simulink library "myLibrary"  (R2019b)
settings: Solver=VariableStepAuto  StartTime=0.0  StopTime=10.0  RelTol=1e-3
undefined symbols (not defined in the file or in its folder): batt_delay, Calculation, cap_1ph, cap_3ph, Complex, Current, Dynamic, EV, ev_charger, EV_ID, ev_num, gcbh, Iabc, Load, max_charge_1ph, max_charge_3ph, max_disch_1ph, max_disch_3ph, MV_LV_transf, myLibrary, phase, Phase, Phasor, rated_1ph, rated_3ph, Single, SoC_init, SPDL, sps_rtmsupport, Tr_capacity, Tstep, Vabc, Vnom, yes
libraries: powerlib x163, $bdroot x13, spsVIMeasurementModel x3, simulink x2, powerlib_meascontrol x1
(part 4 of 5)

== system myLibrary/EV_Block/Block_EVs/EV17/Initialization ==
  Constant : Constant  Value=207.85
  Constant1 : Constant  Value=-120
  Constant2 : Constant  Value=-207.85
  Constant3 : Constant  Value=-120
  Constant4 : Constant  Value=0
  Constant5 : Constant  Value=240
  Constant6 : Constant  Value=Phase
  Data Type Conversion : DataTypeConversion  OutDataTypeStr=double
  Demux : Demux  Outputs=2
  If : If  IfExpression=u1 == 1  ElseIfExpressions=u1 == 2
  If Action Subsystem : Subsystem  TreatAsAtomicUnit=on
  If Action Subsystem1 : Subsystem  TreatAsAtomicUnit=on
  If Action Subsystem2 : Subsystem  TreatAsAtomicUnit=on
  Logical Operator : Logic  Operator=NOT  AllPortsSameDT=off  OutDataTypeStr=boolean
  Mux : Mux  Inputs=2
  Real-Imag to Complex : RealImagToComplex
  Real-Imag to Complex1 : RealImagToComplex
  Real-Imag to Complex2 : RealImagToComplex
  Switch : Switch  Criteria=u2 > Threshold
  Switch1 : Switch  Criteria=u2 > Threshold
  Out1 : Outport  VectorParamsAs1DForOutWhenUnconnected=off
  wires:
  Data Type Conversion/1 -> Mux/2
  [control] -> Demux/1
  Logical Operator/1 -> Data Type Conversion/1
  If Action Subsystem/1(Out1) -> Mux/1
  Mux/1 -> [control]
  If Action Subsystem2/1(Out1) -> Logical Operator/1
  Demux/2 -> Switch1/2
  Demux/1 -> Switch/2
  If/3 -> If Action Subsystem2/Action
  If/2 -> If Action Subsystem1/Action
  If/1 -> If Action Subsystem/Action
  Constant6/1 -> If/1
  Switch1/1 -> Out1/1
  Real-Imag to Complex2/1 -> Switch1/3
  Switch/1 -> Switch1/1
  Real-Imag to Complex1/1 -> Switch/3
  Real-Imag to Complex/1 -> Switch/1
  Constant4/1 -> Real-Imag to Complex2/1
  Constant5/1 -> Real-Imag to Complex2/2
  Constant2/1 -> Real-Imag to Complex1/1
  Constant3/1 -> Real-Imag to Complex1/2
  Constant/1 -> Real-Imag to Complex/1
  Constant1/1 -> Real-Imag to Complex/2

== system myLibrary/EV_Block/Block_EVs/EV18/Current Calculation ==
  Vp : Inport
  Constant : Constant  Commented=on  Value=2060
  Constant1 : Constant  Commented=on  Value=600
  Demux : Demux  Outputs=2
  Divide : Product  Inputs=*/
  From Workspace : FromWorkspace  VariableName=Load_Profile  SampleTime=0  OutputAfterFinalValue=Holding final value
  Gain : Gain  Gain=2
  Math Function : Math  Operator=conj
  Real-Imag to Complex : RealImagToComplex
  Isignal : Outport  VectorParamsAs1DForOutWhenUnconnected=off
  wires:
  Demux/2 -> Real-Imag to Complex/2
  Demux/1 -> Real-Imag to Complex/1
  Math Function/1 -> Isignal/1
  Divide/1 -> Math Function/1
  Gain/1 -> Divide/1
  Vp/1 -> Divide/2
  Real-Imag to Complex/1 -> Gain/1
  From Workspace/1 -> Demux/1

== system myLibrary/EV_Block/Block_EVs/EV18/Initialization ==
  Constant : Constant  Value=207.85
  Constant1 : Constant  Value=-120
  Constant2 : Constant  Value=-207.85
  Constant3 : Constant  Value=-120
  Constant4 : Constant  Value=0
  Constant5 : Constant  Value=240
  Constant6 : Constant  Value=Phase
  Data Type Conversion : DataTypeConversion  OutDataTypeStr=double
  Demux : Demux  Outputs=2
  If : If  IfExpression=u1 == 1  ElseIfExpressions=u1 == 2
  If Action Subsystem : Subsystem  TreatAsAtomicUnit=on
  If Action Subsystem1 : Subsystem  TreatAsAtomicUnit=on
  If Action Subsystem2 : Subsystem  TreatAsAtomicUnit=on
  Logical Operator : Logic  Operator=NOT  AllPortsSameDT=off  OutDataTypeStr=boolean
  Mux : Mux  Inputs=2
  Real-Imag to Complex : RealImagToComplex
  Real-Imag to Complex1 : RealImagToComplex
  Real-Imag to Complex2 : RealImagToComplex
  Switch : Switch  Criteria=u2 > Threshold
  Switch1 : Switch  Criteria=u2 > Threshold
  Out1 : Outport  VectorParamsAs1DForOutWhenUnconnected=off
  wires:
  Data Type Conversion/1 -> Mux/2
  [control] -> Demux/1
  Logical Operator/1 -> Data Type Conversion/1
  If Action Subsystem/1(Out1) -> Mux/1
  Mux/1 -> [control]
  If Action Subsystem2/1(Out1) -> Logical Operator/1
  Demux/2 -> Switch1/2
  Demux/1 -> Switch/2
  If/3 -> If Action Subsystem2/Action
  If/2 -> If Action Subsystem1/Action
  If/1 -> If Action Subsystem/Action
  Constant6/1 -> If/1
  Switch1/1 -> Out1/1
  Real-Imag to Complex2/1 -> Switch1/3
  Switch/1 -> Switch1/1
  Real-Imag to Complex1/1 -> Switch/3
  Real-Imag to Complex/1 -> Switch/1
  Constant4/1 -> Real-Imag to Complex2/1
  Constant5/1 -> Real-Imag to Complex2/2
  Constant2/1 -> Real-Imag to Complex1/1
  Constant3/1 -> Real-Imag to Complex1/2
  Constant/1 -> Real-Imag to Complex/1
  Constant1/1 -> Real-Imag to Complex/2

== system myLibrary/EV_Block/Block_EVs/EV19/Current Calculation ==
  Vp : Inport
  Constant : Constant  Commented=on  Value=2060
  Constant1 : Constant  Commented=on  Value=600
  Demux : Demux  Outputs=2
  Divide : Product  Inputs=*/
  From Workspace : FromWorkspace  VariableName=Load_Profile  SampleTime=0  OutputAfterFinalValue=Holding final value
  Gain : Gain  Gain=2
  Math Function : Math  Operator=conj
  Real-Imag to Complex : RealImagToComplex
  Isignal : Outport  VectorParamsAs1DForOutWhenUnconnected=off
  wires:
  Demux/2 -> Real-Imag to Complex/2
  Demux/1 -> Real-Imag to Complex/1
  Math Function/1 -> Isignal/1
  Divide/1 -> Math Function/1
  Gain/1 -> Divide/1
  Vp/1 -> Divide/2
  Real-Imag to Complex/1 -> Gain/1
  From Workspace/1 -> Demux/1

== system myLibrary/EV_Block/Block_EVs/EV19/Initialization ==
  Constant : Constant  Value=207.85
  Constant1 : Constant  Value=-120
  Constant2 : Constant  Value=-207.85
  Constant3 : Constant  Value=-120
  Constant4 : Constant  Value=0
  Constant5 : Constant  Value=240
  Constant6 : Constant  Value=Phase
  Data Type Conversion : DataTypeConversion  OutDataTypeStr=double
  Demux : Demux  Outputs=2
  If : If  IfExpression=u1 == 1  ElseIfExpressions=u1 == 2
  If Action Subsystem : Subsystem  TreatAsAtomicUnit=on
  If Action Subsystem1 : Subsystem  TreatAsAtomicUnit=on
  If Action Subsystem2 : Subsystem  TreatAsAtomicUnit=on
  Logical Operator : Logic  Operator=NOT  AllPortsSameDT=off  OutDataTypeStr=boolean
  Mux : Mux  Inputs=2
  Real-Imag to Complex : RealImagToComplex
  Real-Imag to Complex1 : RealImagToComplex
  Real-Imag to Complex2 : RealImagToComplex
  Switch : Switch  Criteria=u2 > Threshold
  Switch1 : Switch  Criteria=u2 > Threshold
  Out1 : Outport  VectorParamsAs1DForOutWhenUnconnected=off
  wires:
  Data Type Conversion/1 -> Mux/2
  [control] -> Demux/1
  Logical Operator/1 -> Data Type Conversion/1
  If Action Subsystem/1(Out1) -> Mux/1
  Mux/1 -> [control]
  If Action Subsystem2/1(Out1) -> Logical Operator/1
  Demux/2 -> Switch1/2
  Demux/1 -> Switch/2
  If/3 -> If Action Subsystem2/Action
  If/2 -> If Action Subsystem1/Action
  If/1 -> If Action Subsystem/Action
  Constant6/1 -> If/1
  Switch1/1 -> Out1/1
  Real-Imag to Complex2/1 -> Switch1/3
  Switch/1 -> Switch1/1
  Real-Imag to Complex1/1 -> Switch/3
  Real-Imag to Complex/1 -> Switch/1
  Constant4/1 -> Real-Imag to Complex2/1
  Constant5/1 -> Real-Imag to Complex2/2
  Constant2/1 -> Real-Imag to Complex1/1
  Constant3/1 -> Real-Imag to Complex1/2
  Constant/1 -> Real-Imag to Complex/1
  Constant1/1 -> Real-Imag to Complex/2

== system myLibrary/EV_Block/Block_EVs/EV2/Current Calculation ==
  Vp : Inport
  Constant : Constant  Commented=on  Value=2060
  Constant1 : Constant  Commented=on  Value=600
  Demux : Demux  Outputs=2
  Divide : Product  Inputs=*/
  From Workspace : FromWorkspace  VariableName=Load_Profile  SampleTime=0  OutputAfterFinalValue=Holding final value
  Gain : Gain  Gain=2
  Math Function : Math  Operator=conj
  Real-Imag to Complex : RealImagToComplex
  Isignal : Outport  VectorParamsAs1DForOutWhenUnconnected=off
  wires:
  Demux/2 -> Real-Imag to Complex/2
  Demux/1 -> Real-Imag to Complex/1
  Math Function/1 -> Isignal/1
  Divide/1 -> Math Function/1
  Gain/1 -> Divide/1
  Vp/1 -> Divide/2
  Real-Imag to Complex/1 -> Gain/1
  From Workspace/1 -> Demux/1

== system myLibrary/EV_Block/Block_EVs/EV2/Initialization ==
  Constant : Constant  Value=207.85
  Constant1 : Constant  Value=-120
  Constant2 : Constant  Value=-207.85
  Constant3 : Constant  Value=-120
  Constant4 : Constant  Value=0
  Constant5 : Constant  Value=240
  Constant6 : Constant  Value=Phase
  Data Type Conversion : DataTypeConversion  OutDataTypeStr=double
  Demux : Demux  Outputs=2
  If : If  IfExpression=u1 == 1  ElseIfExpressions=u1 == 2
  If Action Subsystem : Subsystem  TreatAsAtomicUnit=on
  If Action Subsystem1 : Subsystem  TreatAsAtomicUnit=on
  If Action Subsystem2 : Subsystem  TreatAsAtomicUnit=on
  Logical Operator : Logic  Operator=NOT  AllPortsSameDT=off  OutDataTypeStr=boolean
  Mux : Mux  Inputs=2
  Real-Imag to Complex : RealImagToComplex
  Real-Imag to Complex1 : RealImagToComplex
  Real-Imag to Complex2 : RealImagToComplex
  Switch : Switch  Criteria=u2 > Threshold
  Switch1 : Switch  Criteria=u2 > Threshold
  Out1 : Outport  VectorParamsAs1DForOutWhenUnconnected=off
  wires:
  Data Type Conversion/1 -> Mux/2
  [control] -> Demux/1
  Logical Operator/1 -> Data Type Conversion/1
  If Action Subsystem/1(Out1) -> Mux/1
  Mux/1 -> [control]
  If Action Subsystem2/1(Out1) -> Logical Operator/1
  Demux/2 -> Switch1/2
  Demux/1 -> Switch/2
  If/3 -> If Action Subsystem2/Action
  If/2 -> If Action Subsystem1/Action
  If/1 -> If Action Subsystem/Action
  Constant6/1 -> If/1
  Switch1/1 -> Out1/1
  Real-Imag to Complex2/1 -> Switch1/3
  Switch/1 -> Switch1/1
  Real-Imag to Complex1/1 -> Switch/3
  Real-Imag to Complex/1 -> Switch/1
  Constant4/1 -> Real-Imag to Complex2/1
  Constant5/1 -> Real-Imag to Complex2/2
  Constant2/1 -> Real-Imag to Complex1/1
  Constant3/1 -> Real-Imag to Complex1/2
  Constant/1 -> Real-Imag to Complex/1
  Constant1/1 -> Real-Imag to Complex/2

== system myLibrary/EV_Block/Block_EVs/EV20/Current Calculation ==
  Vp : Inport
  Constant : Constant  Commented=on  Value=2060
  Constant1 : Constant  Commented=on  Value=600
  Demux : Demux  Outputs=2
  Divide : Product  Inputs=*/
  From Workspace : FromWorkspace  VariableName=Load_Profile  SampleTime=0  OutputAfterFinalValue=Holding final value
  Gain : Gain  Gain=2
  Math Function : Math  Operator=conj
  Real-Imag to Complex : RealImagToComplex
  Isignal : Outport  VectorParamsAs1DForOutWhenUnconnected=off
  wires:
  Demux/2 -> Real-Imag to Complex/2
  Demux/1 -> Real-Imag to Complex/1
  Math Function/1 -> Isignal/1
  Divide/1 -> Math Function/1
  Gain/1 -> Divide/1
  Vp/1 -> Divide/2
  Real-Imag to Complex/1 -> Gain/1
  From Workspace/1 -> Demux/1

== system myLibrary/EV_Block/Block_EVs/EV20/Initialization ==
  Constant : Constant  Value=207.85
  Constant1 : Constant  Value=-120
  Constant2 : Constant  Value=-207.85
  Constant3 : Constant  Value=-120
  Constant4 : Constant  Value=0
  Constant5 : Constant  Value=240
  Constant6 : Constant  Value=Phase
  Data Type Conversion : DataTypeConversion  OutDataTypeStr=double
  Demux : Demux  Outputs=2
  If : If  IfExpression=u1 == 1  ElseIfExpressions=u1 == 2
  If Action Subsystem : Subsystem  TreatAsAtomicUnit=on
  If Action Subsystem1 : Subsystem  TreatAsAtomicUnit=on
  If Action Subsystem2 : Subsystem  TreatAsAtomicUnit=on
  Logical Operator : Logic  Operator=NOT  AllPortsSameDT=off  OutDataTypeStr=boolean
  Mux : Mux  Inputs=2
  Real-Imag to Complex : RealImagToComplex
  Real-Imag to Complex1 : RealImagToComplex
  Real-Imag to Complex2 : RealImagToComplex
  Switch : Switch  Criteria=u2 > Threshold
  Switch1 : Switch  Criteria=u2 > Threshold
  Out1 : Outport  VectorParamsAs1DForOutWhenUnconnected=off
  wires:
  Data Type Conversion/1 -> Mux/2
  [control] -> Demux/1
  Logical Operator/1 -> Data Type Conversion/1
  If Action Subsystem/1(Out1) -> Mux/1
  Mux/1 -> [control]
  If Action Subsystem2/1(Out1) -> Logical Operator/1
  Demux/2 -> Switch1/2
  Demux/1 -> Switch/2
  If/3 -> If Action Subsystem2/Action
  If/2 -> If Action Subsystem1/Action
  If/1 -> If Action Subsystem/Action
  Constant6/1 -> If/1
  Switch1/1 -> Out1/1
  Real-Imag to Complex2/1 -> Switch1/3
  Switch/1 -> Switch1/1
  Real-Imag to Complex1/1 -> Switch/3
  Real-Imag to Complex/1 -> Switch/1
  Constant4/1 -> Real-Imag to Complex2/1
  Constant5/1 -> Real-Imag to Complex2/2
  Constant2/1 -> Real-Imag to Complex1/1
  Constant3/1 -> Real-Imag to Complex1/2
  Constant/1 -> Real-Imag to Complex/1
  Constant1/1 -> Real-Imag to Complex/2

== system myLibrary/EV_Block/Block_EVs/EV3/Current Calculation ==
  Vp : Inport
  Constant : Constant  Commented=on  Value=2060
  Constant1 : Constant  Commented=on  Value=600
  Demux : Demux  Outputs=2
  Divide : Product  Inputs=*/
  From Workspace : FromWorkspace  VariableName=Load_Profile  SampleTime=0  OutputAfterFinalValue=Holding final value
  Gain : Gain  Gain=2
  Math Function : Math  Operator=conj
  Real-Imag to Complex : RealImagToComplex
  Isignal : Outport  VectorParamsAs1DForOutWhenUnconnected=off
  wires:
  Demux/2 -> Real-Imag to Complex/2
  Demux/1 -> Real-Imag to Complex/1
  Math Function/1 -> Isignal/1
  Divide/1 -> Math Function/1
  Gain/1 -> Divide/1
  Vp/1 -> Divide/2
  Real-Imag to Complex/1 -> Gain/1
  From Workspace/1 -> Demux/1

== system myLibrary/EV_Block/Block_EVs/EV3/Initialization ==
  Constant : Constant  Value=207.85
  Constant1 : Constant  Value=-120
  Constant2 : Constant  Value=-207.85
  Constant3 : Constant  Value=-120
  Constant4 : Constant  Value=0
  Constant5 : Constant  Value=240
  Constant6 : Constant  Value=Phase
  Data Type Conversion : DataTypeConversion  OutDataTypeStr=double
  Demux : Demux  Outputs=2
  If : If  IfExpression=u1 == 1  ElseIfExpressions=u1 == 2
  If Action Subsystem : Subsystem  TreatAsAtomicUnit=on
  If Action Subsystem1 : Subsystem  TreatAsAtomicUnit=on
  If Action Subsystem2 : Subsystem  TreatAsAtomicUnit=on
  Logical Operator : Logic  Operator=NOT  AllPortsSameDT=off  OutDataTypeStr=boolean
  Mux : Mux  Inputs=2
  Real-Imag to Complex : RealImagToComplex
  Real-Imag to Complex1 : RealImagToComplex
  Real-Imag to Complex2 : RealImagToComplex
  Switch : Switch  Criteria=u2 > Threshold
  Switch1 : Switch  Criteria=u2 > Threshold
  Out1 : Outport  VectorParamsAs1DForOutWhenUnconnected=off
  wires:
  Data Type Conversion/1 -> Mux/2
  [control] -> Demux/1
  Logical Operator/1 -> Data Type Conversion/1
  If Action Subsystem/1(Out1) -> Mux/1
  Mux/1 -> [control]
  If Action Subsystem2/1(Out1) -> Logical Operator/1
  Demux/2 -> Switch1/2
  Demux/1 -> Switch/2
  If/3 -> If Action Subsystem2/Action
  If/2 -> If Action Subsystem1/Action
  If/1 -> If Action Subsystem/Action
  Constant6/1 -> If/1
  Switch1/1 -> Out1/1
  Real-Imag to Complex2/1 -> Switch1/3
  Switch/1 -> Switch1/1
  Real-Imag to Complex1/1 -> Switch/3
  Real-Imag to Complex/1 -> Switch/1
  Constant4/1 -> Real-Imag to Complex2/1
  Constant5/1 -> Real-Imag to Complex2/2
  Constant2/1 -> Real-Imag to Complex1/1
  Constant3/1 -> Real-Imag to Complex1/2
  Constant/1 -> Real-Imag to Complex/1
  Constant1/1 -> Real-Imag to Complex/2

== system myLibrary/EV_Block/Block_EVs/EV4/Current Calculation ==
  Vp : Inport
  Constant : Constant  Commented=on  Value=2060
  Constant1 : Constant  Commented=on  Value=600
  Demux : Demux  Outputs=2
  Divide : Product  Inputs=*/
  From Workspace : FromWorkspace  VariableName=Load_Profile  SampleTime=0  OutputAfterFinalValue=Holding final value
  Gain : Gain  Gain=2
  Math Function : Math  Operator=conj
  Real-Imag to Complex : RealImagToComplex
  Isignal : Outport  VectorParamsAs1DForOutWhenUnconnected=off
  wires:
  Demux/2 -> Real-Imag to Complex/2
  Demux/1 -> Real-Imag to Complex/1
  Math Function/1 -> Isignal/1
  Divide/1 -> Math Function/1
  Gain/1 -> Divide/1
  Vp/1 -> Divide/2
  Real-Imag to Complex/1 -> Gain/1
  From Workspace/1 -> Demux/1

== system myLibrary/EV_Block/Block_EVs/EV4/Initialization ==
  Constant : Constant  Value=207.85
  Constant1 : Constant  Value=-120
  Constant2 : Constant  Value=-207.85
  Constant3 : Constant  Value=-120
  Constant4 : Constant  Value=0
  Constant5 : Constant  Value=240
  Constant6 : Constant  Value=Phase
  Data Type Conversion : DataTypeConversion  OutDataTypeStr=double
  Demux : Demux  Outputs=2
  If : If  IfExpression=u1 == 1  ElseIfExpressions=u1 == 2
  If Action Subsystem : Subsystem  TreatAsAtomicUnit=on
  If Action Subsystem1 : Subsystem  TreatAsAtomicUnit=on
  If Action Subsystem2 : Subsystem  TreatAsAtomicUnit=on
  Logical Operator : Logic  Operator=NOT  AllPortsSameDT=off  OutDataTypeStr=boolean
  Mux : Mux  Inputs=2
  Real-Imag to Complex : RealImagToComplex
  Real-Imag to Complex1 : RealImagToComplex
  Real-Imag to Complex2 : RealImagToComplex
  Switch : Switch  Criteria=u2 > Threshold
  Switch1 : Switch  Criteria=u2 > Threshold
  Out1 : Outport  VectorParamsAs1DForOutWhenUnconnected=off
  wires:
  Data Type Conversion/1 -> Mux/2
  [control] -> Demux/1
  Logical Operator/1 -> Data Type Conversion/1
  If Action Subsystem/1(Out1) -> Mux/1
  Mux/1 -> [control]
  If Action Subsystem2/1(Out1) -> Logical Operator/1
  Demux/2 -> Switch1/2
  Demux/1 -> Switch/2
  If/3 -> If Action Subsystem2/Action
  If/2 -> If Action Subsystem1/Action
  If/1 -> If Action Subsystem/Action
  Constant6/1 -> If/1
  Switch1/1 -> Out1/1
  Real-Imag to Complex2/1 -> Switch1/3
  Switch/1 -> Switch1/1
  Real-Imag to Complex1/1 -> Switch/3
  Real-Imag to Complex/1 -> Switch/1
  Constant4/1 -> Real-Imag to Complex2/1
  Constant5/1 -> Real-Imag to Complex2/2
  Constant2/1 -> Real-Imag to Complex1/1
  Constant3/1 -> Real-Imag to Complex1/2
  Constant/1 -> Real-Imag to Complex/1
  Constant1/1 -> Real-Imag to Complex/2

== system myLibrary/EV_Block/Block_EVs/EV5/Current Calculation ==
  Vp : Inport
  Constant : Constant  Commented=on  Value=2060
  Constant1 : Constant  Commented=on  Value=600
  Demux : Demux  Outputs=2
  Divide : Product  Inputs=*/
  From Workspace : FromWorkspace  VariableName=Load_Profile  SampleTime=0  OutputAfterFinalValue=Holding final value
  Gain : Gain  Gain=2
  Math Function : Math  Operator=conj
  Real-Imag to Complex : RealImagToComplex
  Isignal : Outport  VectorParamsAs1DForOutWhenUnconnected=off
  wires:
  Demux/2 -> Real-Imag to Complex/2
  Demux/1 -> Real-Imag to Complex/1
  Math Function/1 -> Isignal/1
  Divide/1 -> Math Function/1
  Gain/1 -> Divide/1
  Vp/1 -> Divide/2
  Real-Imag to Complex/1 -> Gain/1
  From Workspace/1 -> Demux/1

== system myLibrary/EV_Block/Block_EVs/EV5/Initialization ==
  Constant : Constant  Value=207.85
  Constant1 : Constant  Value=-120
  Constant2 : Constant  Value=-207.85
  Constant3 : Constant  Value=-120
  Constant4 : Constant  Value=0
  Constant5 : Constant  Value=240
  Constant6 : Constant  Value=Phase
  Data Type Conversion : DataTypeConversion  OutDataTypeStr=double
  Demux : Demux  Outputs=2
  If : If  IfExpression=u1 == 1  ElseIfExpressions=u1 == 2
  If Action Subsystem : Subsystem  TreatAsAtomicUnit=on
  If Action Subsystem1 : Subsystem  TreatAsAtomicUnit=on
  If Action Subsystem2 : Subsystem  TreatAsAtomicUnit=on
  Logical Operator : Logic  Operator=NOT  AllPortsSameDT=off  OutDataTypeStr=boolean
  Mux : Mux  Inputs=2
  Real-Imag to Complex : RealImagToComplex
  Real-Imag to Complex1 : RealImagToComplex
  Real-Imag to Complex2 : RealImagToComplex
  Switch : Switch  Criteria=u2 > Threshold
  Switch1 : Switch  Criteria=u2 > Threshold
  Out1 : Outport  VectorParamsAs1DForOutWhenUnconnected=off
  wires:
  Data Type Conversion/1 -> Mux/2
  [control] -> Demux/1
  Logical Operator/1 -> Data Type Conversion/1
  If Action Subsystem/1(Out1) -> Mux/1
  Mux/1 -> [control]
  If Action Subsystem2/1(Out1) -> Logical Operator/1
  Demux/2 -> Switch1/2
  Demux/1 -> Switch/2
  If/3 -> If Action Subsystem2/Action
  If/2 -> If Action Subsystem1/Action
  If/1 -> If Action Subsystem/Action
  Constant6/1 -> If/1
  Switch1/1 -> Out1/1
  Real-Imag to Complex2/1 -> Switch1/3
  Switch/1 -> Switch1/1
  Real-Imag to Complex1/1 -> Switch/3
  Real-Imag to Complex/1 -> Switch/1
  Constant4/1 -> Real-Imag to Complex2/1
  Constant5/1 -> Real-Imag to Complex2/2
  Constant2/1 -> Real-Imag to Complex1/1
  Constant3/1 -> Real-Imag to Complex1/2
  Constant/1 -> Real-Imag to Complex/1
  Constant1/1 -> Real-Imag to Complex/2

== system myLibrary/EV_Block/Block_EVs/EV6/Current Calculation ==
  Vp : Inport
  Constant : Constant  Commented=on  Value=2060
  Constant1 : Constant  Commented=on  Value=600
  Demux : Demux  Outputs=2
  Divide : Product  Inputs=*/
  From Workspace : FromWorkspace  VariableName=Load_Profile  SampleTime=0  OutputAfterFinalValue=Holding final value
  Gain : Gain  Gain=2
  Math Function : Math  Operator=conj
  Real-Imag to Complex : RealImagToComplex
  Isignal : Outport  VectorParamsAs1DForOutWhenUnconnected=off
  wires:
  Demux/2 -> Real-Imag to Complex/2
  Demux/1 -> Real-Imag to Complex/1
  Math Function/1 -> Isignal/1
  Divide/1 -> Math Function/1
  Gain/1 -> Divide/1
  Vp/1 -> Divide/2
  Real-Imag to Complex/1 -> Gain/1
  From Workspace/1 -> Demux/1

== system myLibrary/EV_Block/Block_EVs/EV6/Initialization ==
  Constant : Constant  Value=207.85
  Constant1 : Constant  Value=-120
  Constant2 : Constant  Value=-207.85
  Constant3 : Constant  Value=-120
  Constant4 : Constant  Value=0
  Constant5 : Constant  Value=240
  Constant6 : Constant  Value=Phase
  Data Type Conversion : DataTypeConversion  OutDataTypeStr=double
  Demux : Demux  Outputs=2
  If : If  IfExpression=u1 == 1  ElseIfExpressions=u1 == 2
  If Action Subsystem : Subsystem  TreatAsAtomicUnit=on
  If Action Subsystem1 : Subsystem  TreatAsAtomicUnit=on
  If Action Subsystem2 : Subsystem  TreatAsAtomicUnit=on
  Logical Operator : Logic  Operator=NOT  AllPortsSameDT=off  OutDataTypeStr=boolean
  Mux : Mux  Inputs=2
  Real-Imag to Complex : RealImagToComplex
  Real-Imag to Complex1 : RealImagToComplex
  Real-Imag to Complex2 : RealImagToComplex
  Switch : Switch  Criteria=u2 > Threshold
  Switch1 : Switch  Criteria=u2 > Threshold
  Out1 : Outport  VectorParamsAs1DForOutWhenUnconnected=off
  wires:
  Data Type Conversion/1 -> Mux/2
  [control] -> Demux/1
  Logical Operator/1 -> Data Type Conversion/1
  If Action Subsystem/1(Out1) -> Mux/1
  Mux/1 -> [control]
  If Action Subsystem2/1(Out1) -> Logical Operator/1
  Demux/2 -> Switch1/2
  Demux/1 -> Switch/2
  If/3 -> If Action Subsystem2/Action
  If/2 -> If Action Subsystem1/Action
  If/1 -> If Action Subsystem/Action
  Constant6/1 -> If/1
  Switch1/1 -> Out1/1
  Real-Imag to Complex2/1 -> Switch1/3
  Switch/1 -> Switch1/1
  Real-Imag to Complex1/1 -> Switch/3
  Real-Imag to Complex/1 -> Switch/1
  Constant4/1 -> Real-Imag to Complex2/1
  Constant5/1 -> Real-Imag to Complex2/2
  Constant2/1 -> Real-Imag to Complex1/1
  Constant3/1 -> Real-Imag to Complex1/2
  Constant/1 -> Real-Imag to Complex/1
  Constant1/1 -> Real-Imag to Complex/2

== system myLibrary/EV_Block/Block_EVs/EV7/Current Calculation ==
  Vp : Inport
  Constant : Constant  Commented=on  Value=2060
  Constant1 : Constant  Commented=on  Value=600
  Demux : Demux  Outputs=2
  Divide : Product  Inputs=*/
  From Workspace : FromWorkspace  VariableName=Load_Profile  SampleTime=0  OutputAfterFinalValue=Holding final value
  Gain : Gain  Gain=2
  Math Function : Math  Operator=conj
  Real-Imag to Complex : RealImagToComplex
  Isignal : Outport  VectorParamsAs1DForOutWhenUnconnected=off
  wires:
  Demux/2 -> Real-Imag to Complex/2
  Demux/1 -> Real-Imag to Complex/1
  Math Function/1 -> Isignal/1
  Divide/1 -> Math Function/1
  Gain/1 -> Divide/1
  Vp/1 -> Divide/2
  Real-Imag to Complex/1 -> Gain/1
  From Workspace/1 -> Demux/1

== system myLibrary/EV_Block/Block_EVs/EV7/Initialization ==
  Constant : Constant  Value=207.85
  Constant1 : Constant  Value=-120
  Constant2 : Constant  Value=-207.85
  Constant3 : Constant  Value=-120
  Constant4 : Constant  Value=0
  Constant5 : Constant  Value=240
  Constant6 : Constant  Value=Phase
  Data Type Conversion : DataTypeConversion  OutDataTypeStr=double
  Demux : Demux  Outputs=2
  If : If  IfExpression=u1 == 1  ElseIfExpressions=u1 == 2
  If Action Subsystem : Subsystem  TreatAsAtomicUnit=on
  If Action Subsystem1 : Subsystem  TreatAsAtomicUnit=on
  If Action Subsystem2 : Subsystem  TreatAsAtomicUnit=on
  Logical Operator : Logic  Operator=NOT  AllPortsSameDT=off  OutDataTypeStr=boolean
  Mux : Mux  Inputs=2
  Real-Imag to Complex : RealImagToComplex
  Real-Imag to Complex1 : RealImagToComplex
  Real-Imag to Complex2 : RealImagToComplex
  Switch : Switch  Criteria=u2 > Threshold
  Switch1 : Switch  Criteria=u2 > Threshold
  Out1 : Outport  VectorParamsAs1DForOutWhenUnconnected=off
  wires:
  Data Type Conversion/1 -> Mux/2
  [control] -> Demux/1
  Logical Operator/1 -> Data Type Conversion/1
  If Action Subsystem/1(Out1) -> Mux/1
  Mux/1 -> [control]
  If Action Subsystem2/1(Out1) -> Logical Operator/1
  Demux/2 -> Switch1/2
  Demux/1 -> Switch/2
  If/3 -> If Action Subsystem2/Action
  If/2 -> If Action Subsystem1/Action
  If/1 -> If Action Subsystem/Action
  Constant6/1 -> If/1
  Switch1/1 -> Out1/1
  Real-Imag to Complex2/1 -> Switch1/3
  Switch/1 -> Switch1/1
  Real-Imag to Complex1/1 -> Switch/3
  Real-Imag to Complex/1 -> Switch/1
  Constant4/1 -> Real-Imag to Complex2/1
  Constant5/1 -> Real-Imag to Complex2/2
  Constant2/1 -> Real-Imag to Complex1/1
  Constant3/1 -> Real-Imag to Complex1/2
  Constant/1 -> Real-Imag to Complex/1
  Constant1/1 -> Real-Imag to Complex/2

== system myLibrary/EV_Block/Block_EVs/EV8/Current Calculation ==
  Vp : Inport
  Constant : Constant  Commented=on  Value=2060
  Constant1 : Constant  Commented=on  Value=600
  Demux : Demux  Outputs=2
  Divide : Product  Inputs=*/
  From Workspace : FromWorkspace  VariableName=Load_Profile  SampleTime=0  OutputAfterFinalValue=Holding final value
  Gain : Gain  Gain=2
  Math Function : Math  Operator=conj
  Real-Imag to Complex : RealImagToComplex
  Isignal : Outport  VectorParamsAs1DForOutWhenUnconnected=off
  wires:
  Demux/2 -> Real-Imag to Complex/2
  Demux/1 -> Real-Imag to Complex/1
  Math Function/1 -> Isignal/1
  Divide/1 -> Math Function/1
  Gain/1 -> Divide/1
  Vp/1 -> Divide/2
  Real-Imag to Complex/1 -> Gain/1
  From Workspace/1 -> Demux/1

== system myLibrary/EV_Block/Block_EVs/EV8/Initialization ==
  Constant : Constant  Value=207.85
  Constant1 : Constant  Value=-120
  Constant2 : Constant  Value=-207.85
  Constant3 : Constant  Value=-120
  Constant4 : Constant  Value=0
  Constant5 : Constant  Value=240
  Constant6 : Constant  Value=Phase
  Data Type Conversion : DataTypeConversion  OutDataTypeStr=double
  Demux : Demux  Outputs=2
  If : If  IfExpression=u1 == 1  ElseIfExpressions=u1 == 2
  If Action Subsystem : Subsystem  TreatAsAtomicUnit=on
  If Action Subsystem1 : Subsystem  TreatAsAtomicUnit=on
  If Action Subsystem2 : Subsystem  TreatAsAtomicUnit=on
  Logical Operator : Logic  Operator=NOT  AllPortsSameDT=off  OutDataTypeStr=boolean
  Mux : Mux  Inputs=2
  Real-Imag to Complex : RealImagToComplex
  Real-Imag to Complex1 : RealImagToComplex
  Real-Imag to Complex2 : RealImagToComplex
  Switch : Switch  Criteria=u2 > Threshold
  Switch1 : Switch  Criteria=u2 > Threshold
  Out1 : Outport  VectorParamsAs1DForOutWhenUnconnected=off
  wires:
  Data Type Conversion/1 -> Mux/2
  [control] -> Demux/1
  Logical Operator/1 -> Data Type Conversion/1
  If Action Subsystem/1(Out1) -> Mux/1
  Mux/1 -> [control]
  If Action Subsystem2/1(Out1) -> Logical Operator/1
  Demux/2 -> Switch1/2
  Demux/1 -> Switch/2
  If/3 -> If Action Subsystem2/Action
  If/2 -> If Action Subsystem1/Action
  If/1 -> If Action Subsystem/Action
  Constant6/1 -> If/1
  Switch1/1 -> Out1/1
  Real-Imag to Complex2/1 -> Switch1/3
  Switch/1 -> Switch1/1
  Real-Imag to Complex1/1 -> Switch/3
  Real-Imag to Complex/1 -> Switch/1
  Constant4/1 -> Real-Imag to Complex2/1
  Constant5/1 -> Real-Imag to Complex2/2
  Constant2/1 -> Real-Imag to Complex1/1
  Constant3/1 -> Real-Imag to Complex1/2
  Constant/1 -> Real-Imag to Complex/1
  Constant1/1 -> Real-Imag to Complex/2

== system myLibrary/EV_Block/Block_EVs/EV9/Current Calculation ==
  Vp : Inport
  Constant : Constant  Commented=on  Value=2060
  Constant1 : Constant  Commented=on  Value=600
  Demux : Demux  Outputs=2
  Divide : Product  Inputs=*/
  From Workspace : FromWorkspace  VariableName=Load_Profile  SampleTime=0  OutputAfterFinalValue=Holding final value
  Gain : Gain  Gain=2
  Math Function : Math  Operator=conj
  Real-Imag to Complex : RealImagToComplex
  Isignal : Outport  VectorParamsAs1DForOutWhenUnconnected=off
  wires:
  Demux/2 -> Real-Imag to Complex/2
  Demux/1 -> Real-Imag to Complex/1
  Math Function/1 -> Isignal/1
  Divide/1 -> Math Function/1
  Gain/1 -> Divide/1
  Vp/1 -> Divide/2
  Real-Imag to Complex/1 -> Gain/1
  From Workspace/1 -> Demux/1

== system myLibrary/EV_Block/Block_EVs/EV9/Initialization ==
  Constant : Constant  Value=207.85
  Constant1 : Constant  Value=-120
  Constant2 : Constant  Value=-207.85
  Constant3 : Constant  Value=-120
  Constant4 : Constant  Value=0
  Constant5 : Constant  Value=240
  Constant6 : Constant  Value=Phase
  Data Type Conversion : DataTypeConversion  OutDataTypeStr=double
  Demux : Demux  Outputs=2
  If : If  IfExpression=u1 == 1  ElseIfExpressions=u1 == 2
  If Action Subsystem : Subsystem  TreatAsAtomicUnit=on
  If Action Subsystem1 : Subsystem  TreatAsAtomicUnit=on
  If Action Subsystem2 : Subsystem  TreatAsAtomicUnit=on
  Logical Operator : Logic  Operator=NOT  AllPortsSameDT=off  OutDataTypeStr=boolean
  Mux : Mux  Inputs=2
  Real-Imag to Complex : RealImagToComplex
  Real-Imag to Complex1 : RealImagToComplex
  Real-Imag to Complex2 : RealImagToComplex
  Switch : Switch  Criteria=u2 > Threshold
  Switch1 : Switch  Criteria=u2 > Threshold
  Out1 : Outport  VectorParamsAs1DForOutWhenUnconnected=off
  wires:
  Data Type Conversion/1 -> Mux/2
  [control] -> Demux/1
  Logical Operator/1 -> Data Type Conversion/1
  If Action Subsystem/1(Out1) -> Mux/1
  Mux/1 -> [control]
  If Action Subsystem2/1(Out1) -> Logical Operator/1
  Demux/2 -> Switch1/2
  Demux/1 -> Switch/2
  If/3 -> If Action Subsystem2/Action
  If/2 -> If Action Subsystem1/Action
  If/1 -> If Action Subsystem/Action
  Constant6/1 -> If/1
  Switch1/1 -> Out1/1
  Real-Imag to Complex2/1 -> Switch1/3
  Switch/1 -> Switch1/1
  Real-Imag to Complex1/1 -> Switch/3
  Real-Imag to Complex/1 -> Switch/1
  Constant4/1 -> Real-Imag to Complex2/1
  Constant5/1 -> Real-Imag to Complex2/2
  Constant2/1 -> Real-Imag to Complex1/1
  Constant3/1 -> Real-Imag to Complex1/2
  Constant/1 -> Real-Imag to Complex/1
  Constant1/1 -> Real-Imag to Complex/2

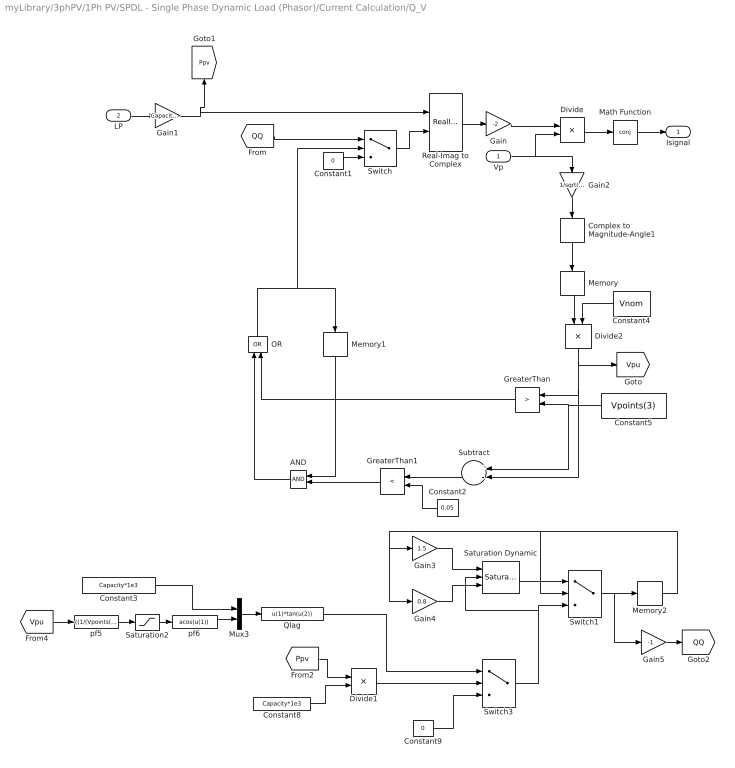
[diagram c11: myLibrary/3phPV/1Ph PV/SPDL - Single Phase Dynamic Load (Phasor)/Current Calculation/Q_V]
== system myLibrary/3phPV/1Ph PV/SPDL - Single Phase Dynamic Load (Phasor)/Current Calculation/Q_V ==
  Vp : Inport
  LP : Inport  Port=2
  AND : Logic  IconShape=distinctive  AllPortsSameDT=off  OutDataTypeStr=boolean
  Complex to Magnitude-Angle1 : ComplexToMagnitudeAngle  Output=Magnitude
  Constant1 : Constant  Value=0
  Constant2 : Constant  Value=0.05
  Constant3 : Constant  Value=Capacity*1e3
  Constant4 : Constant  Value=Vnom
  Constant5 : Constant  Value=Vpoints(3)
  Constant8 : Constant  Value=Capacity*1e3
  Constant9 : Constant  Value=0
  Divide : Product  Inputs=*/
  Divide1 : Product  Inputs=*/
  Divide2 : Product  Inputs=*/
  Gain : Gain  Gain=-2
  Gain1 : Gain  Gain=Capacity*1000
  Gain2 : Gain  Gain=1/sqrt(2)
  Gain3 : Gain  Gain=1.5
  Gain4 : Gain  Gain=0.8
  Gain5 : Gain  Gain=-1
  GreaterThan : RelationalOperator  Operator=>  OutDataTypeStr=boolean  RndMeth=Simplest
  GreaterThan1 : RelationalOperator  Operator=<  OutDataTypeStr=boolean  RndMeth=Simplest
  Math Function : Math  Operator=conj
  Memory : Memory  InitialCondition=Vnom
  Memory1 : Memory
  Memory2 : Memory
  Mux3 : Mux  Inputs=2
  OR : Logic  Operator=OR  IconShape=distinctive  AllPortsSameDT=off  OutDataTypeStr=boolean
  Qlag : Fcn  Expr=u(1)*tan(u(2))
  Real-Imag to Complex : RealImagToComplex
  Saturation Dynamic : simulink/Discontinuities/Saturation Dynamic  OutMin=[]  OutMax=[]  OutDataTypeStr=Inherit: Same as second input  OutDataType=fixdt(1, 16)  OutScaling=2^-10  DoSatur=off
  Saturation2 : Saturate  UpperLimit=1  LowerLimit=0.9
  Subtract : Sum  Inputs=+-
  Switch : Switch  Threshold=0.5
  Switch1 : Switch  Threshold=100
  Switch3 : Switch  Threshold=0.01
  pf5 : Fcn  Expr=((1/(Vpoints(3)-Vpoints(4)))*((1-pf_V)*u(1)+pf_V*Vpoints(3)-Vpoints(4)))
  pf6 : Fcn  Expr=acos(u(1))
  Isignal : Outport  VectorParamsAs1DForOutWhenUnconnected=off
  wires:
  Vp/1 -> Gain2/1, Divide/2
  Divide/1 -> Math Function/1
  Real-Imag to Complex/1 -> Gain/1
  Gain/1 -> Divide/1
  Math Function/1 -> Isignal/1
  Constant1/1 -> Switch/3
  Switch/1 -> Real-Imag to Complex/2
  Gain1/1 -> Real-Imag to Complex/1, [Ppv]
  LP/1 -> Gain1/1
  Constant4/1 -> Divide2/2
  Constant5/1 -> GreaterThan/2, Subtract/1
  Complex to Magnitude-Angle1/1 -> Memory/1
  Divide2/1 -> GreaterThan/1, Subtract/2, [Vpu]
  Gain2/1 -> Complex to Magnitude-Angle1/1
  Memory/1 -> Divide2/1
  Subtract/1 -> GreaterThan1/1
  Constant2/1 -> GreaterThan1/2
  GreaterThan1/1 -> AND/2
  Memory1/1 -> AND/1
  AND/1 -> OR/1
  GreaterThan/1 -> OR/2
  OR/1 -> Switch/2, Memory1/1
  [QQ] -> Switch/1
  Constant8/1 -> Divide1/2
  Saturation Dynamic/1 -> Switch1/1
  Gain3/1 -> Saturation Dynamic/1
  [Vpu] -> pf5/1
  Constant3/1 -> Mux3/1
  [Ppv] -> Divide1/1
  Mux3/1 -> Qlag/1
  pf6/1 -> Mux3/2
  Constant9/1 -> Switch3/3
  Divide1/1 -> Switch3/2
  Qlag/1 -> Switch3/1
  Gain4/1 -> Saturation Dynamic/3
  pf5/1 -> Saturation2/1
  Saturation2/1 -> pf6/1
  Switch3/1 -> Switch1/3, Saturation Dynamic/2
  Gain5/1 -> [QQ]
  Memory2/1 -> Gain4/1, Gain3/1, Switch1/2
  Switch1/1 -> Gain5/1, Memory2/1

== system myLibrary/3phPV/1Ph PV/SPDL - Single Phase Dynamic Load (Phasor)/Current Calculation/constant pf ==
  Vp : Inport
  LP : Inport  Port=2
  Constant1 : Constant  Value=0
  Constant10 : Constant  Value=pf
  Divide : Product  Inputs=*/
  Gain : Gain  Gain=-2
  Gain1 : Gain  Gain=Capacity*1000
  Math Function : Math  Operator=conj
  Mux : Mux  Inputs=2
  Q : Fcn  Expr=-u(1)*tan(acos(u(2)))
  Real-Imag to Complex : RealImagToComplex
  Switch : Switch  Threshold=0.1
  Isignal : Outport  VectorParamsAs1DForOutWhenUnconnected=off
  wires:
  Gain1/1 -> Real-Imag to Complex/1, Mux/1
  Vp/1 -> Divide/2
  LP/1 -> Switch/2, Gain1/1
  Constant10/1 -> Mux/2
  Divide/1 -> Math Function/1
  Q/1 -> Switch/1
  Real-Imag to Complex/1 -> Gain/1
  Gain/1 -> Divide/1
  Mux/1 -> Q/1
  Math Function/1 -> Isignal/1
  Constant1/1 -> Switch/3
  Switch/1 -> Real-Imag to Complex/2

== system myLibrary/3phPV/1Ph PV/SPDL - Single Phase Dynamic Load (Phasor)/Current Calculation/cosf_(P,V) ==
  Vp : Inport
  LP : Inport  Port=2
  Complex to Magnitude-Angle1 : ComplexToMagnitudeAngle  Output=Magnitude
  Constant1 : Constant  Value=0
  Constant4 : Constant  Value=Vnom
  Divide : Product  Inputs=*/
  Divide2 : Product  Inputs=*/
  Gain : Gain  Gain=-2
  Gain1 : Gain  Gain=Capacity*1000
  Gain2 : Gain  Gain=1/sqrt(2)
  Math Function : Math  Operator=conj
  Memory : Memory  InitialCondition=Vnom
  Mux : Mux  Inputs=2
  Mux1 : Mux  Inputs=2
  Q : Fcn  Expr=-u(1)*tan(u(2))
  Real-Imag to Complex : RealImagToComplex
  Saturation : Saturate  UpperLimit=1  LowerLimit=pfend
  Switch : Switch  Threshold=Pstart
  pf1 : Fcn  Expr=acos((1/(Pstart-1))*(u(1)*(1-u(2))+Pstart*u(2)-1))
  pf2 : Fcn  Expr=(((1-pfend)/(Vstart-1.1))*(u(1)-Vstart)+1)
  Isignal : Outport  VectorParamsAs1DForOutWhenUnconnected=off
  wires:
  Vp/1 -> Gain2/1, Divide/2
  Divide/1 -> Math Function/1
  Real-Imag to Complex/1 -> Gain/1
  Gain/1 -> Divide/1
  Math Function/1 -> Isignal/1
  Constant1/1 -> Switch/3
  Switch/1 -> Real-Imag to Complex/2
  Gain1/1 -> Real-Imag to Complex/1, Mux/1
  Mux/1 -> Q/1
  LP/1 -> Switch/2, Mux1/1, Gain1/1
  Q/1 -> Switch/1
  pf1/1 -> Mux/2
  Constant4/1 -> Divide2/2
  Complex to Magnitude-Angle1/1 -> Memory/1
  Gain2/1 -> Complex to Magnitude-Angle1/1
  Memory/1 -> Divide2/1
  Divide2/1 -> pf2/1
  pf2/1 -> Saturation/1
  Mux1/1 -> pf1/1
  Saturation/1 -> Mux1/2

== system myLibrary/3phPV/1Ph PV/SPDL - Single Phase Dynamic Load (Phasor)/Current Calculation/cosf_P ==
  Vp : Inport
  LP : Inport  Port=2
  Constant1 : Constant  Value=0
  Divide : Product  Inputs=*/
  Gain : Gain  Gain=-2
  Gain1 : Gain  Gain=Capacity*1000
  Math Function : Math  Operator=conj
  Mux : Mux  Inputs=2
  Q : Fcn  Expr=-u(1)*tan(u(2))
  Real-Imag to Complex : RealImagToComplex
  Switch : Switch  Threshold=Pstart
  pf1 : Fcn  Expr=acos((1/(Pstart-1))*(u(1)*(1-pfend)+Pstart*pfend-1))
  Isignal : Outport  VectorParamsAs1DForOutWhenUnconnected=off
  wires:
  Vp/1 -> Divide/2
  Divide/1 -> Math Function/1
  Real-Imag to Complex/1 -> Gain/1
  Gain/1 -> Divide/1
  Math Function/1 -> Isignal/1
  Constant1/1 -> Switch/3
  Switch/1 -> Real-Imag to Complex/2
  Gain1/1 -> Mux/1, Real-Imag to Complex/1
  Mux/1 -> Q/1
  LP/1 -> Switch/2, pf1/1, Gain1/1
  Q/1 -> Switch/1
  pf1/1 -> Mux/2

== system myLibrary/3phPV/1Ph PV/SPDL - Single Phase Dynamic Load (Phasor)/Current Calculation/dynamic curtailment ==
  Vp : Inport
  Pin : Inport  Port=2
  Complex to Magnitude-Angle1 : ComplexToMagnitudeAngle  Output=Magnitude
  Constant1 : Constant  Value=0.1
  Constant4 : Constant  Value=Vnom
  Divide2 : Product  Inputs=*/
  Gain2 : Gain  Gain=1/sqrt(2)
  Gain3 : Gain  Gain=1.2
  Gain4 : Gain  Gain=0.8
  Less Than : RelationalOperator  Operator=<  OutDataTypeStr=boolean  RndMeth=Simplest
  Less Than1 : RelationalOperator  Operator=<  OutDataTypeStr=boolean  RndMeth=Simplest
  Memory : Memory  InitialCondition=Vnom
  Memory1 : Memory
  OR : Logic  Operator=OR  IconShape=distinctive  AllPortsSameDT=off  OutDataTypeStr=boolean
  Saturation : Saturate  UpperLimit=1  LowerLimit=Pmin
  Saturation Dynamic : simulink/Discontinuities/Saturation Dynamic  OutMin=[]  OutMax=[]  OutDataTypeStr=Inherit: Same as second input  OutDataType=fixdt(1, 16)  OutScaling=2^-10  DoSatur=off
  Switch : Switch  Criteria=u2 > Threshold
  curtailment : Fcn  Expr=((Pmin-1)/(Vend-Vstart))*(u(1)-Vstart)+1
  Pout : Outport  VectorParamsAs1DForOutWhenUnconnected=off
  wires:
  Vp/1 -> Gain2/1
  Constant4/1 -> Divide2/2
  Complex to Magnitude-Angle1/1 -> Memory/1
  Gain2/1 -> Complex to Magnitude-Angle1/1
  Memory/1 -> Divide2/1
  curtailment/1 -> Saturation/1
  Divide2/1 -> curtailment/1
  Pin/1 -> Less Than1/1, Less Than/1, Switch/1
  Switch/1 -> Pout/1, Memory1/1
  Gain3/1 -> Saturation Dynamic/1
  Gain4/1 -> Saturation Dynamic/3
  Memory1/1 -> Gain4/1, Gain3/1
  Saturation/1 -> Saturation Dynamic/2
  Saturation Dynamic/1 -> Less Than/2, Switch/3
  OR/1 -> Switch/2
  Less Than/1 -> OR/1
  Less Than1/1 -> OR/2
  Constant1/1 -> Less Than1/2

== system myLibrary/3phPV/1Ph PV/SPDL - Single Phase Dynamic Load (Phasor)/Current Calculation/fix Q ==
  Vp : Inport
  LP : Inport  Port=2
  Constant1 : Constant  Value=0
  Constant2 : Constant  Value=-Capacity*1000*tan(acos(pf))
  Divide : Product  Inputs=*/
  Gain : Gain  Gain=-2
  Gain1 : Gain  Gain=Capacity*1000
  Math Function : Math  Operator=conj
  Real-Imag to Complex : RealImagToComplex
  Switch : Switch  Threshold=0.1
  Isignal : Outport  VectorParamsAs1DForOutWhenUnconnected=off
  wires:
  Vp/1 -> Divide/2
  Divide/1 -> Math Function/1
  Real-Imag to Complex/1 -> Gain/1
  Gain/1 -> Divide/1
  Math Function/1 -> Isignal/1
  Constant1/1 -> Switch/3
  Switch/1 -> Real-Imag to Complex/2
  Gain1/1 -> Real-Imag to Complex/1
  LP/1 -> Switch/2, Gain1/1
  Constant2/1 -> Switch/1

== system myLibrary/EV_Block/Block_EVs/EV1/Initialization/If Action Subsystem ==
  Action Port : ActionPort
  Constant : Constant
  Out1 : Outport  VectorParamsAs1DForOutWhenUnconnected=off
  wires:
  Constant/1 -> Out1/1

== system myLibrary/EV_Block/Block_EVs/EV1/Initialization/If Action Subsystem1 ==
  Action Port : ActionPort
  Constant : Constant
  Out1 : Outport  VectorParamsAs1DForOutWhenUnconnected=off
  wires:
  Constant/1 -> Out1/1

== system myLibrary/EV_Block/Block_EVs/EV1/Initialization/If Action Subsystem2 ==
  Action Port : ActionPort
  Constant : Constant
  Out1 : Outport  VectorParamsAs1DForOutWhenUnconnected=off
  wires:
  Constant/1 -> Out1/1

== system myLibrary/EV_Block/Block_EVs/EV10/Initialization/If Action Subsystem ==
  Action Port : ActionPort
  Constant : Constant
  Out1 : Outport  VectorParamsAs1DForOutWhenUnconnected=off
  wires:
  Constant/1 -> Out1/1

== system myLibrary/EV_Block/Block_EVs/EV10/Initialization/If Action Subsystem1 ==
  Action Port : ActionPort
  Constant : Constant
  Out1 : Outport  VectorParamsAs1DForOutWhenUnconnected=off
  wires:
  Constant/1 -> Out1/1

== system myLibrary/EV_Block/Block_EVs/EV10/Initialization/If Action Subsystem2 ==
  Action Port : ActionPort
  Constant : Constant
  Out1 : Outport  VectorParamsAs1DForOutWhenUnconnected=off
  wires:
  Constant/1 -> Out1/1

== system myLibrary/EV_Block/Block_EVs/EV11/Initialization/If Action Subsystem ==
  Action Port : ActionPort
  Constant : Constant
  Out1 : Outport  VectorParamsAs1DForOutWhenUnconnected=off
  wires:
  Constant/1 -> Out1/1

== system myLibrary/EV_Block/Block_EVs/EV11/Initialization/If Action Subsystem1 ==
  Action Port : ActionPort
  Constant : Constant
  Out1 : Outport  VectorParamsAs1DForOutWhenUnconnected=off
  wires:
  Constant/1 -> Out1/1

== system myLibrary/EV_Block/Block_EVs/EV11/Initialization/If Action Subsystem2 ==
  Action Port : ActionPort
  Constant : Constant
  Out1 : Outport  VectorParamsAs1DForOutWhenUnconnected=off
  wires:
  Constant/1 -> Out1/1

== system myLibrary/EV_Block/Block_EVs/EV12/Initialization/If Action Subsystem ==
  Action Port : ActionPort
  Constant : Constant
  Out1 : Outport  VectorParamsAs1DForOutWhenUnconnected=off
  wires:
  Constant/1 -> Out1/1

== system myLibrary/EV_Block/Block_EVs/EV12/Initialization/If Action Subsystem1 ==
  Action Port : ActionPort
  Constant : Constant
  Out1 : Outport  VectorParamsAs1DForOutWhenUnconnected=off
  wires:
  Constant/1 -> Out1/1

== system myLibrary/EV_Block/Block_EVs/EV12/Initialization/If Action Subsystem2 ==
  Action Port : ActionPort
  Constant : Constant
  Out1 : Outport  VectorParamsAs1DForOutWhenUnconnected=off
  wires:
  Constant/1 -> Out1/1

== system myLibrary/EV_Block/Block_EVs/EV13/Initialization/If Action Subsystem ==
  Action Port : ActionPort
  Constant : Constant
  Out1 : Outport  VectorParamsAs1DForOutWhenUnconnected=off
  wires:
  Constant/1 -> Out1/1

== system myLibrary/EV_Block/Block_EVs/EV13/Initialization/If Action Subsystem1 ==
  Action Port : ActionPort
  Constant : Constant
  Out1 : Outport  VectorParamsAs1DForOutWhenUnconnected=off
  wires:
  Constant/1 -> Out1/1

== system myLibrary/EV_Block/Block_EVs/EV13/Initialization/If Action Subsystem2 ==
  Action Port : ActionPort
  Constant : Constant
  Out1 : Outport  VectorParamsAs1DForOutWhenUnconnected=off
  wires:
  Constant/1 -> Out1/1

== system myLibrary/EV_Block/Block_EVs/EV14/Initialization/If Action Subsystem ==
  Action Port : ActionPort
  Constant : Constant
  Out1 : Outport  VectorParamsAs1DForOutWhenUnconnected=off
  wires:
  Constant/1 -> Out1/1

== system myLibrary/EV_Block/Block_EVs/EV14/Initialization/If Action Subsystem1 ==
  Action Port : ActionPort
  Constant : Constant
  Out1 : Outport  VectorParamsAs1DForOutWhenUnconnected=off
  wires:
  Constant/1 -> Out1/1

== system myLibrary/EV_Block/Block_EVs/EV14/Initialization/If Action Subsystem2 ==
  Action Port : ActionPort
  Constant : Constant
  Out1 : Outport  VectorParamsAs1DForOutWhenUnconnected=off
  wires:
  Constant/1 -> Out1/1

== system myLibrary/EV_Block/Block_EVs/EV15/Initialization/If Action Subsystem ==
  Action Port : ActionPort
  Constant : Constant
  Out1 : Outport  VectorParamsAs1DForOutWhenUnconnected=off
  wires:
  Constant/1 -> Out1/1

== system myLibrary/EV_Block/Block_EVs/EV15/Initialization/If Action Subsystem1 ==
  Action Port : ActionPort
  Constant : Constant
  Out1 : Outport  VectorParamsAs1DForOutWhenUnconnected=off
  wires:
  Constant/1 -> Out1/1

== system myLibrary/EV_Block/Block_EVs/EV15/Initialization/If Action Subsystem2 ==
  Action Port : ActionPort
  Constant : Constant
  Out1 : Outport  VectorParamsAs1DForOutWhenUnconnected=off
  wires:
  Constant/1 -> Out1/1

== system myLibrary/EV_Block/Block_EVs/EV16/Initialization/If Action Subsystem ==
  Action Port : ActionPort
  Constant : Constant
  Out1 : Outport  VectorParamsAs1DForOutWhenUnconnected=off
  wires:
  Constant/1 -> Out1/1

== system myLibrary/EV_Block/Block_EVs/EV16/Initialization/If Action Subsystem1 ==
  Action Port : ActionPort
  Constant : Constant
  Out1 : Outport  VectorParamsAs1DForOutWhenUnconnected=off
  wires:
  Constant/1 -> Out1/1

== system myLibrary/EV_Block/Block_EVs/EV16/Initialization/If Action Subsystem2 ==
  Action Port : ActionPort
  Constant : Constant
  Out1 : Outport  VectorParamsAs1DForOutWhenUnconnected=off
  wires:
  Constant/1 -> Out1/1

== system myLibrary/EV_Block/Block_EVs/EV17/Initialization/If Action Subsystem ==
  Action Port : ActionPort
  Constant : Constant
  Out1 : Outport  VectorParamsAs1DForOutWhenUnconnected=off
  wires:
  Constant/1 -> Out1/1

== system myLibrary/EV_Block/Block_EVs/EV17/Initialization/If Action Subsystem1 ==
  Action Port : ActionPort
  Constant : Constant
  Out1 : Outport  VectorParamsAs1DForOutWhenUnconnected=off
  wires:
  Constant/1 -> Out1/1

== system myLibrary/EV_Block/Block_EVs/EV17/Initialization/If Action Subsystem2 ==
  Action Port : ActionPort
  Constant : Constant
  Out1 : Outport  VectorParamsAs1DForOutWhenUnconnected=off
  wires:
  Constant/1 -> Out1/1

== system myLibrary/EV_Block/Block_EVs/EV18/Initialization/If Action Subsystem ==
  Action Port : ActionPort
  Constant : Constant
  Out1 : Outport  VectorParamsAs1DForOutWhenUnconnected=off
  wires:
  Constant/1 -> Out1/1

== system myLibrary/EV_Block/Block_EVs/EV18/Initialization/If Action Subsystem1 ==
  Action Port : ActionPort
  Constant : Constant
  Out1 : Outport  VectorParamsAs1DForOutWhenUnconnected=off
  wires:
  Constant/1 -> Out1/1

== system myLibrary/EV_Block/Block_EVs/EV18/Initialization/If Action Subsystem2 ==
  Action Port : ActionPort
  Constant : Constant
  Out1 : Outport  VectorParamsAs1DForOutWhenUnconnected=off
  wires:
  Constant/1 -> Out1/1

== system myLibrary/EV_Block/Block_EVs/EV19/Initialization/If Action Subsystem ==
  Action Port : ActionPort
  Constant : Constant
  Out1 : Outport  VectorParamsAs1DForOutWhenUnconnected=off
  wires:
  Constant/1 -> Out1/1

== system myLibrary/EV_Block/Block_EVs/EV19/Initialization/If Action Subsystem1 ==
  Action Port : ActionPort
  Constant : Constant
  Out1 : Outport  VectorParamsAs1DForOutWhenUnconnected=off
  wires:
  Constant/1 -> Out1/1

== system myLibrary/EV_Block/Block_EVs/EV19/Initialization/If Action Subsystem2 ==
  Action Port : ActionPort
  Constant : Constant
  Out1 : Outport  VectorParamsAs1DForOutWhenUnconnected=off
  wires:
  Constant/1 -> Out1/1

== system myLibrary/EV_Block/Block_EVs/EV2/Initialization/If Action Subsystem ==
  Action Port : ActionPort
  Constant : Constant
  Out1 : Outport  VectorParamsAs1DForOutWhenUnconnected=off
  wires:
  Constant/1 -> Out1/1

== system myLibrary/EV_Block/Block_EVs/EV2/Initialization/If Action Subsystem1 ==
  Action Port : ActionPort
  Constant : Constant
  Out1 : Outport  VectorParamsAs1DForOutWhenUnconnected=off
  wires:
  Constant/1 -> Out1/1

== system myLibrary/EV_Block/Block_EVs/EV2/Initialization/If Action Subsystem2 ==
  Action Port : ActionPort
  Constant : Constant
  Out1 : Outport  VectorParamsAs1DForOutWhenUnconnected=off
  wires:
  Constant/1 -> Out1/1

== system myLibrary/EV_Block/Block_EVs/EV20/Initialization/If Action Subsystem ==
  Action Port : ActionPort
  Constant : Constant
  Out1 : Outport  VectorParamsAs1DForOutWhenUnconnected=off
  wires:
  Constant/1 -> Out1/1

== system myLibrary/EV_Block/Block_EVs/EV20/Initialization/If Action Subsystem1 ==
  Action Port : ActionPort
  Constant : Constant
  Out1 : Outport  VectorParamsAs1DForOutWhenUnconnected=off
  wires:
  Constant/1 -> Out1/1

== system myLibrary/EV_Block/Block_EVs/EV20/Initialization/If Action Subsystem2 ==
  Action Port : ActionPort
  Constant : Constant
  Out1 : Outport  VectorParamsAs1DForOutWhenUnconnected=off
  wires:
  Constant/1 -> Out1/1

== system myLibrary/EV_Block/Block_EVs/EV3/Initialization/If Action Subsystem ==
  Action Port : ActionPort
  Constant : Constant
  Out1 : Outport  VectorParamsAs1DForOutWhenUnconnected=off
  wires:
  Constant/1 -> Out1/1

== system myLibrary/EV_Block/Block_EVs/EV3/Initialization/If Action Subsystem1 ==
  Action Port : ActionPort
  Constant : Constant
  Out1 : Outport  VectorParamsAs1DForOutWhenUnconnected=off
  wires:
  Constant/1 -> Out1/1

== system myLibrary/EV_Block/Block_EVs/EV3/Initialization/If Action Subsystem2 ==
  Action Port : ActionPort
  Constant : Constant
  Out1 : Outport  VectorParamsAs1DForOutWhenUnconnected=off
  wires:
  Constant/1 -> Out1/1

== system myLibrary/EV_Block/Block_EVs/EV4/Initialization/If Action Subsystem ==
  Action Port : ActionPort
  Constant : Constant
  Out1 : Outport  VectorParamsAs1DForOutWhenUnconnected=off
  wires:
  Constant/1 -> Out1/1

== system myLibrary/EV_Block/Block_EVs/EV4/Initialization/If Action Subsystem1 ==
  Action Port : ActionPort
  Constant : Constant
  Out1 : Outport  VectorParamsAs1DForOutWhenUnconnected=off
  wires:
  Constant/1 -> Out1/1

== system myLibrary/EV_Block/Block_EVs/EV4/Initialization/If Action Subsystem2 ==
  Action Port : ActionPort
  Constant : Constant
  Out1 : Outport  VectorParamsAs1DForOutWhenUnconnected=off
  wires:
  Constant/1 -> Out1/1
